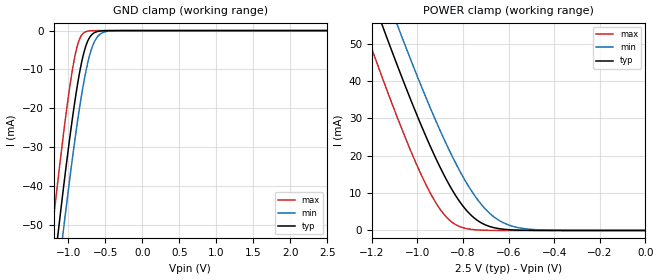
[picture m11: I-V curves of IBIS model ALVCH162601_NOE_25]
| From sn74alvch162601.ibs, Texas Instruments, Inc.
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[Model]   ALVCH162601_NOE_25
Model_type  Input
Vinl=0.7
Vinh=1.7
| variable   typ   min   max
C_comp   2.08pF   1.80pF   2.36pF
[Temperature Range]   40   100   -40
| Ambient temperature   25   85   -40
[Voltage range]   2.5   2.3   2.7
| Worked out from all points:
|   GND clamp passes 1 mA (typ) near -0.68 V on its own axis
|   POWER clamp passes 1 mA (typ) near -0.68 V on its own axis
[GND Clamp]
| ALVCH162601_NOE_25
|   Voltage   I(typ)   I(min)   I(max)
-2.5V     -300mA     -309.4mA   -288.3mA
-1.22V    -65.92mA   -76.78mA   -51.96mA
-1.15V    -54.2mA    -65.07mA   -40.19mA
-1.125V   -50.1mA    -60.96mA   -36.1mA
-1.07V    -41.27mA   -52.08mA   -27.39mA
-980mV    -27.63mA   -38.14mA   -14.46mA
-910mV    -18.08mA   -28.05mA   -6.523mA
-845mV    -10.58mA   -19.54mA   -2.069mA
-780mV    -5.041mA   -12.24mA   -440.8uA
-655mV    -630uA     -3.209mA   -15.41uA
-485mV    -21.18uA   -229.3uA   -148.8nA
2.5V      1.112nA    1.808uA    4.19pA
[POWER Clamp]
| ALVCH162601_NOE_25
|   Voltage   I(typ)   I(min)   I(max)
-2.5V     300mA      309.4mA    288.3mA
-1.24V    69.32mA    80.17mA    55.39mA
-1.22V    65.92mA    76.78mA    51.96mA
-1.145V   53.37mA    64.25mA    39.37mA
-1.09V    44.44mA    55.28mA    30.51mA
-1.075V   42.06mA    52.87mA    28.16mA
-970mV    26.19mA    36.66mA    13.17mA
-880mV    14.42mA    24mA       4.064mA
-770mV    4.399mA    11.26mA    340.3uA
-665mV    761.4uA    3.659mA    20.23uA
-510mV    35.16uA    347.7uA    294.5nA
-31.15fV  1.112nA    59.61nA    5.15pA
